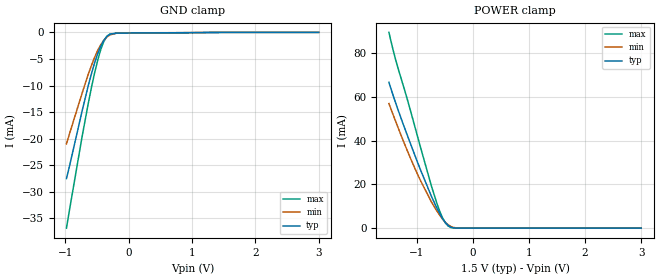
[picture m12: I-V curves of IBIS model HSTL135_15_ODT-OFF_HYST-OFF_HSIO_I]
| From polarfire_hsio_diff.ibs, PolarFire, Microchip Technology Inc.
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|   HSTL135_15_ODT-OFF_HYST-OFF_HSIO_I
[Model]   HSTL135_15_ODT-OFF_HYST-OFF_HSIO_I
Model_type  Input
Vinl =   0.585
Vinh =   0.765
|   typ   min   max
C_comp_pullup   1.335e-12   1.335e-12   1.380e-12
C_comp_pulldown  1.335e-12   1.335e-12   1.380e-12
[Temperature Range]   25   100   -40
[Voltage Range]   1.5   1.425   1.575
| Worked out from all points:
|   GND clamp passes 1 mA (typ) near -0.36 V on its own axis
|   POWER clamp passes 1 mA (typ) near -0.43 V on its own axis
[GND Clamp]
| Voltage   I(typ)   I(min)   I(max)
-984.4mV  -27.52mA   -20.98mA   -36.83mA
-738.3mV  -14.86mA   -11.51mA   -19.71mA
-639.8mV  -10.04mA   -7.906mA   -13.38mA
-590.6mV  -7.836mA   -6.26mA    -10.46mA
-492.2mV  -4.065mA   -3.445mA   -5.32mA
-443mV    -2.601mA   -2.343mA   -3.27mA
-393.7mV  -1.488mA   -1.479mA   -1.705mA
-344.5mV  -752.6uA   -861.2uA   -730.4uA
-295.3mV  -360.6uA   -471.6uA   -308.6uA
-196.9mV  -143.8uA   -162.9uA   -160.9uA
-49.22mV  -116uA     -99.1uA    -145.8uA
3V        0A         0A         0A
[POWER Clamp]
| Voltage   I(typ)   I(min)   I(max)
-1.5V     66.68mA    56.94mA    89.5mA
-1.378V   57.1mA     48.68mA    76.77mA
-1.083V   36.37mA    30mA       50.67mA
-935.2mV  26.53mA    21.65mA    36.81mA
-738.3mV  14.34mA    11.83mA    18.94mA
-590.6mV  6.46mA     5.758mA    7.505mA
-541.4mV  4.304mA    4.076mA    4.577mA
-492.2mV  2.523mA    2.637mA    2.357mA
-443mV    1.219mA    1.504mA    952.6uA
-344.5mV  140.1uA    299.1uA    81.87uA
-196.9mV  20.92uA    25.77uA    23.8uA
3V        0A         0A         0A
